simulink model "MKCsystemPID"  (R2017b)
settings: Solver=ode3  StartTime=0.0  StopTime=T  FixedStep=dt  RelTol=1e-3
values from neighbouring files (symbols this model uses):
  A = 0.01    [para20191204.m]
  c1 = 100    [para20191204.m]
  f = 1*2*pi    (= 6.28318530718)    [para20191204.m]
  k1 = 10    [para20191204.m]
  k2 = 20    [para20191204.m]
  Kd = 0    [para20191204.m]
  Ki = 0    [para20191204.m]
  Kp = 2000    [para20191204.m]
  m1 = 1    [para20191204.m]
  m2 = 0.1    [para20191204.m]

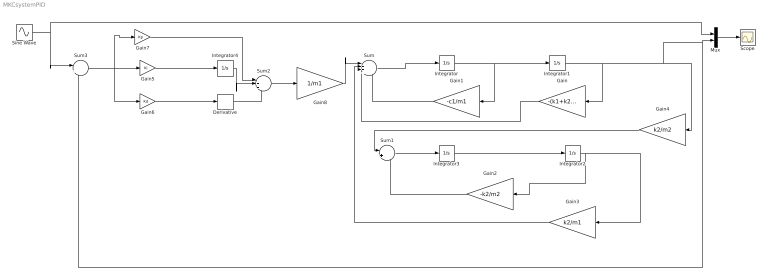
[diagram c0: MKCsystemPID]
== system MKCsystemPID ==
  Derivative : Derivative
  Gain : Gain  Gain=-(k1+k2)/m1
  Gain1 : Gain  Gain=-c1/m1
  Gain2 : Gain  Gain=-k2/m2
  Gain3 : Gain  Gain=k2/m1
  Gain4 : Gain  Gain=k2/m2
  Gain5 : Gain  Gain=Ki
  Gain6 : Gain  Gain=Kd
  Gain7 : Gain  Gain=Kp
  Gain8 : Gain  Gain=1/m1
  Integrator{,1..4} (5 alike) : Integrator
  Mux : Mux  Inputs=2
  Scope : Scope
  Sine Wave : Sin  Amplitude=A  Frequency=f  SampleTime=0
  Sum : Sum  Inputs=|++++
  Sum1 : Sum  Inputs=|++
  Sum2 : Sum  Inputs=|+++
  Sum3 : Sum  Inputs=|+-
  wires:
  Integrator/1 -> Gain1/1, Integrator1/1
  Gain1/1 -> Sum/4
  Integrator1/1 -> Gain/1, Sum3/2, Mux/2, Gain4/1
  Gain4/1 -> Sum1/1
  Sum1/1 -> Integrator3/1
  Integrator3/1 -> Integrator2/1
  Integrator2/1 -> Gain3/1, Gain2/1
  Gain2/1 -> Sum1/2
  Gain/1 -> Sum/3
  Gain3/1 -> Sum/2
  Sum/1 -> Integrator/1
  Gain5/1 -> Integrator4/1
  Gain6/1 -> Derivative/1
  Sine Wave/1 -> Mux/1, Sum3/1
  Sum3/1 -> Gain6/1, Gain5/1, Gain7/1
  Gain7/1 -> Sum2/1
  Integrator4/1 -> Sum2/2
  Derivative/1 -> Sum2/3
  Sum2/1 -> Gain8/1
  Gain8/1 -> Sum/1
  Mux/1 -> Scope/1
